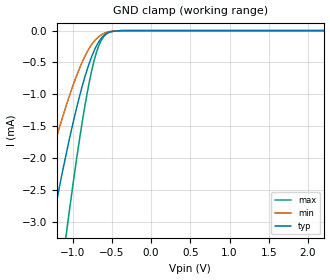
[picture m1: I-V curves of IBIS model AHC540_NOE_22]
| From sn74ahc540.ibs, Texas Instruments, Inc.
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[Model]   AHC540_NOE_22
Model_type  Input
Vinl = 0.5
Vinh = 1.5
| variable   typ   min   max
C_comp   0.68pF   0.62pF   0.73pF
[Temperature Range]   40   100   -40
| Ambient temperature   25   85   -40
[Voltage range]   2.2   2   2.4
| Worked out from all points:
|   GND clamp passes 1 mA (typ) near -0.91 V on its own axis
[GND Clamp]
| AHC540_NOE_22
|   Voltage   I(typ)   I(min)   I(max)
-5V       -39.52mA   -26.01mA   -50.56mA
-1.555V   -5.15mA    -3.294mA   -8.099mA
-1.505V   -4.773mA   -3.047mA   -7.55mA
-1.305V   -3.345mA   -2.108mA   -5.419mA
-1.255V   -3.011mA   -1.888mA   -4.905mA
-1.075V   -1.895mA   -1.152mA   -3.138mA
-910mV    -1.023mA   -586.6uA   -1.69mA
-775mV    -468.5uA   -252.2uA   -732.7uA
-680mV    -204.3uA   -109.6uA   -283.9uA
-565mV    -45.2uA    -27.94uA   -48.8uA
-385mV    -1.717uA   -1.239uA   -925.9nA
2.2V      1.234nA    466.5pA    2.192nA
